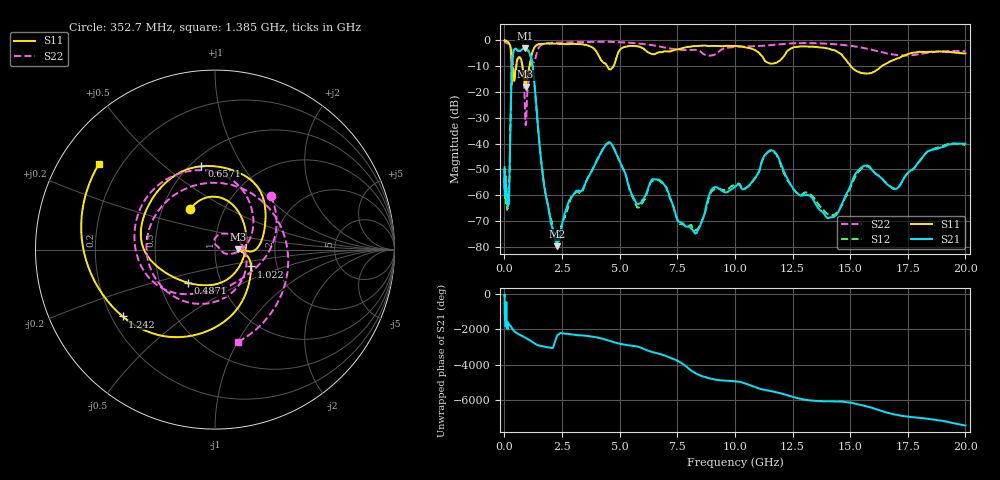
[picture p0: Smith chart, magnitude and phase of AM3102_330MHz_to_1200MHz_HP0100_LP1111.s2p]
! Date/Time: Tue, Sep 11, 2018 5:13 PM
! Network Analyzer: Agilent Technologies E8362B Rev: A.07.50.63
! Sweep from 0.010 to 20.000 GHz, 1601 Points, Sweep Type: LOG
! Power Supply: 4.949 V, 0.001 A
# Hz S DB R 50
!freq MagS11 AngS11 MagS21 AngS21 MagS12 AngS12 MagS22 AngS22
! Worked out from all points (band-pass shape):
!   1601 points, 10 MHz to 20 GHz, reference 50 ohm
!   highest |S21| = -3.02 dB at 886.4 MHz (marker M1); lowest = -79.8 dB at 2.292 GHz (marker M2)
!   |S21| within 3 dB of the highest: 358.2 MHz to 1.138 GHz (779.7 MHz wide, 104 % of centre)
!   lowest |S11| = -17.9 dB at 920.7 MHz (marker M3), VSWR 1.29, Z = 64.5 + j0.293 ohm
!   |S11| at or under -10 dB: 781.2 MHz to 1.088 GHz (307.1 MHz wide, 32.9 % of centre); 4.459 GHz to 4.733 GHz (274.3 MHz wide, 5.97 % of centre); 15.03 GHz to 16.37 GHz (1.346 GHz wide, 8.57 % of centre)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
!   |S22| runs from -32.9 to -0.3 dB; largest |S21 - S12| = 0.013
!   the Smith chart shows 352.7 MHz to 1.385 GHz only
!   S11 on the Smith chart (normalised r, x): 352.7 MHz: 0.69, +0.33; 487.1 MHz: 0.70, -0.27; 657.1 MHz: 0.57, +0.68; 1.022 GHz: 1.47, -0.29; 1.242 GHz: 0.25, -0.31; 1.385 GHz: 0.12, +0.32
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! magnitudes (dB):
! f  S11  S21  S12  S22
! 10 MHz  0.0  -53.8  -48.8  -0.3
! 35.55 MHz  0.0  -56.9  -59.3  -0.6
! 126.4 MHz  -0.4  -61.4  -62.4  -1.1
! 207.2 MHz  -1.2  -59.5  -57.3  -1.4
! 352.7 MHz  -11.6  -6.4  -6.4  -7.3
! 447.2 MHz  -14.9  -3.3  -3.4  -13.2
! 487.1 MHz  -12.5  -3.2  -3.3  -11.6
! 657.1 MHz  -6.5  -4.0  -4.2  -6.4
! 886.4 MHz  -16.7  -3.0  -3.1  -25.2
! 920.7 MHz  -17.9  -3.1  -3.2  -32.8
! 1.022 GHz  -13.1  -3.8  -3.8  -17.9
! 1.242 GHz  -3.9  -11.2  -11.3  -8.4
! 1.385 GHz  -1.9  -25.3  -25.7  -5.5
! 1.59 GHz  -1.4  -46.2  -46.2  -1.8
! 2.292 GHz  -1.3  -79.8  -78.4  -0.8
! 4.479 GHz  -10.3  -39.9  -39.8  -0.5
! 5.652 GHz  -2.1  -61.9  -62.7  -1.0
! 6.675 GHz  -4.7  -54.0  -54.2  -2.2
! 8.227 GHz  -2.2  -74.3  -73.2  -3.6
! 11.58 GHz  -9.0  -42.5  -42.9  -1.8
! 14.07 GHz  -3.2  -68.9  -67.7  -1.3
! 20 GHz  -5.0  -40.1  -40.6  -4.2
